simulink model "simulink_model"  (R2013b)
settings: Solver=ode1  StartTime=0.0  StopTime=inf  FixedStep=0.0001  RelTol=1e-3
PostLoadFcn:
  | , if any(exist('dsrtsu_mdlpostloadfcn', 'file') == [2, 3, 6]), try dsrtsu_mdlpostloadfcn('Execute', bdroot); catch fprintf('Error in PostLoadFcn (dsrtsu_mdlpostloadfcn) for model "%s":\n %s\n', bdroot, lasterr); end, end,
libraries: rtilib1103 x8, simulink x4

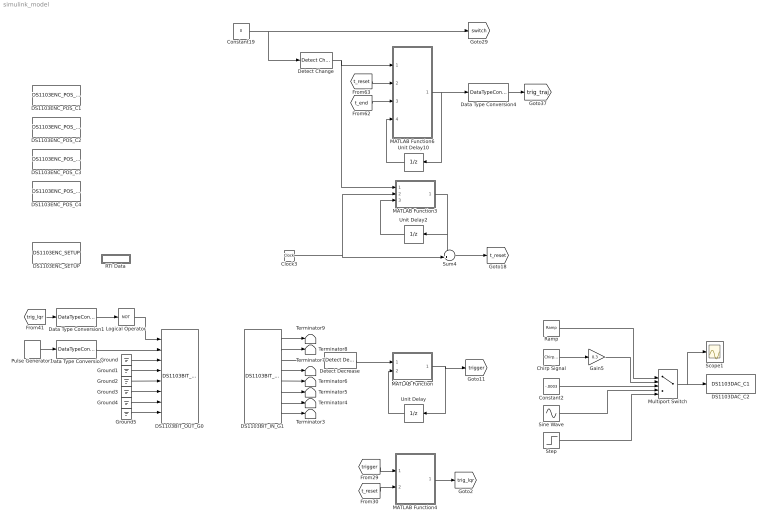
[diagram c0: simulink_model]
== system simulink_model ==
  Chirp Signal : simulink/Sources/Chirp Signal  f1=0.3  T=5  f2=1
  Clock3 : Clock
  Constant19 : Constant  Value=0  OutDataTypeStr=double
  Constant2 : Constant  Value=-.0003  OutDataTypeStr=double
  DS1103BIT_IN_G1 : rtilib1103/DS1103 MASTER PPC/DS1103BIT_IN_G0  GroupNo=1  Reserved1=[]  Reserved2=[]  Reserved3=[]  Reserved4=[]  DialogFcn=gui1103bit_inx  UnitName={ 'DS1103BIT_IN_G'}  UnitValues={ 1 }  DSProperties=struct('RTI',struct('Version',uint32(1),'BlockType',struct('isSLSource',uint8(1),'isSLSink',uint8(0),'isHWSource',uint8(1),'isHWSink',uint8(0),'isSetup',uint8(0),'isInline',uint8(1),'isNonInline',uint8(0),'isInterrupt',uint8(0),'isChannelwise',uint8(0)),'IOBoardType','DS1103MASTER','UnitType','BIT','Identifier','BITIN','DialogType','ML','BlockSet','NONE','SlaveProcessor','NONE'))
  DS1103BIT_OUT_G0 : rtilib1103/DS1103 MASTER PPC/DS1103BIT_OUT_G0  GroupNo=0  InitValue=[0 0 0 0 0 0 0 0]  TermMode=[1 1 1 1 1 1 1 1]  TermValue=[0 0 0 0 0 0 0 0]  Reserved1=[]  Reserved2=[]  Reserved3=[]  Reserved=[]  DialogFcn=gui1103bit_out  UnitName={ 'DS1103BIT_OUT_G'}  UnitValues={ 0 }  DSProperties=struct('RTI',struct('Version',uint32(1),'BlockType',struct('isSLSource',uint8(0),'isSLSink',uint8(1),'isHWSource',uint8(0),'isHWSink',uint8(1),'isSetup',uint8(0),'isInline',uint8(1),'isNonInline',uint8(0),'isInterrupt',uint8(0),'isChannelwise',uint8(0)),'IOBoardType','DS1103MASTER','UnitType','BIT','Identifier','BITOUT','DialogType','ML','BlockSet','NONE','SlaveProcessor','NONE'))
  DS1103DAC_C2 : rtilib1103/DS1103 MASTER PPC/DS1103DAC_C1  ChannelNo=2  InitValue=0  TermMode=1  TermValue=0  Reserved1=[]  Reserved2=[]  Reserved3=[]  Reserved4=[]  DialogFcn=gui1103dac  UnitName={ 'DS1103DAC_C' }  UnitValues={ 2 }  DSProperties=struct('RTI',struct('Version',uint32(1),'BlockType',struct('isSLSource',uint8(0),'isSLSink',uint8(1),'isHWSource',uint8(0),'isHWSink',uint8(1),'isSetup',uint8(0),'isInline',uint8(1),'isNonInline',uint8(0),'isInterrupt',uint8(0),'isChannelwise',uint8(1)),'IOBoardType','DS1103MASTER','UnitType','DAC','Identifier','DAC','DialogType','ML','BlockSet','NONE','SlaveProcessor','NONE'))
  DS1103ENC_POS_C1 : rtilib1103/DS1103 MASTER PPC/DS1103ENC_POS_C1  ChannelNo=1  PosValue=-1024  Reserved1=[]  Reserved2=[]  Reserved3=[]  Reserved4=[]  DialogFcn=gui1103enc_pos  UnitName={ 'DS1103ENC_POS_C' }  UnitValues={ 1 }  DSProperties=struct('RTI',struct('Version',uint32(1),'BlockType',struct('isSLSource',uint8(1),'isSLSink',uint8(0),'isHWSource',uint8(1),'isHWSink',uint8(0),'isSetup',uint8(0),'isInline',uint8(1),'isNonInline',uint8(0),'isInterrupt',uint8(0),'isChannelwise',uint8(1)),'IOBoardType','DS1103MASTER','UnitType','ENC','Identifier','ENCPOSCH','DialogType','ML','BlockSet','NONE','SlaveProcessor','NONE'))
  DS1103ENC_POS_C2 : rtilib1103/DS1103 MASTER PPC/DS1103ENC_POS_C1  ChannelNo=2  PosValue=0  Reserved1=[]  Reserved2=[]  Reserved3=[]  Reserved4=[]  DialogFcn=gui1103enc_pos  UnitName={ 'DS1103ENC_POS_C' }  UnitValues={ 2 }  DSProperties=struct('RTI',struct('Version',uint32(1),'BlockType',struct('isSLSource',uint8(1),'isSLSink',uint8(0),'isHWSource',uint8(1),'isHWSink',uint8(0),'isSetup',uint8(0),'isInline',uint8(1),'isNonInline',uint8(0),'isInterrupt',uint8(0),'isChannelwise',uint8(1)),'IOBoardType','DS1103MASTER','UnitType','ENC','Identifier','ENCPOSCH','DialogType','ML','BlockSet','NONE','SlaveProcessor','NONE'))
  DS1103ENC_POS_C3 : rtilib1103/DS1103 MASTER PPC/DS1103ENC_POS_C1  ChannelNo=3  PosValue=0  Reserved1=[]  Reserved2=[]  Reserved3=[]  Reserved4=[]  DialogFcn=gui1103enc_pos  UnitName={ 'DS1103ENC_POS_C' }  UnitValues={3}  DSProperties=struct('RTI',struct('Version',uint32(1),'BlockType',struct('isSLSource',uint8(1),'isSLSink',uint8(0),'isHWSource',uint8(1),'isHWSink',uint8(0),'isSetup',uint8(0),'isInline',uint8(1),'isNonInline',uint8(0),'isInterrupt',uint8(0),'isChannelwise',uint8(1)),'IOBoardType','DS1103MASTER','UnitType','ENC','Identifier','ENCPOSCH','DialogType','ML','BlockSet','NONE','SlaveProcessor','NONE'))
  DS1103ENC_POS_C4 : rtilib1103/DS1103 MASTER PPC/DS1103ENC_POS_C1  ChannelNo=4  PosValue=0  Reserved1=[]  Reserved2=[]  Reserved3=[]  Reserved4=[]  DialogFcn=gui1103enc_pos  UnitName={ 'DS1103ENC_POS_C' }  UnitValues={ 4 }  DSProperties=struct('RTI',struct('Version',uint32(1),'BlockType',struct('isSLSource',uint8(1),'isSLSink',uint8(0),'isHWSource',uint8(1),'isHWSink',uint8(0),'isSetup',uint8(0),'isInline',uint8(1),'isNonInline',uint8(0),'isInterrupt',uint8(0),'isChannelwise',uint8(1)),'IOBoardType','DS1103MASTER','UnitType','ENC','Identifier','ENCPOSCH','DialogType','ML','BlockSet','NONE','SlaveProcessor','NONE'))
  DS1103ENC_SETUP : rtilib1103/DS1103 MASTER PPC/DS1103ENC_SETUP  EncRange=0  Reserved1=[]  Reserved2=[]  Reserved3=[]  Reserved4=[]  DialogFcn=gui1103enc_setup  UnitName={ 'DS1103ENC_SETUP' }  UnitValues={ [] }  DSProperties=struct('RTI',struct('Version',uint32(1),'BlockType',struct('isSLSource',uint8(0),'isSLSink',uint8(0),'isHWSource',uint8(0),'isHWSink',uint8(0),'isSetup',uint8(0),'isInline',uint8(1),'isNonInline',uint8(0),'isInterrupt',uint8(0),'isChannelwise',uint8(0)),'IOBoardType','DS1103MASTER','UnitType','ENC','Identifier','ENCMASTER','DialogType','ML','BlockSet','NONE','SlaveProcessor','NONE'))
  Data Type Conversion : DataTypeConversion
  Data Type Conversion1 : DataTypeConversion
  Data Type Conversion4 : DataTypeConversion  OutDataTypeStr=boolean
  Detect Change : simulink/Logic and Bit Operations/Detect Change  vinit=0  InputProcessing=Inherited  OutDataTypeStr=boolean
  Detect Decrease : simulink/Logic and Bit Operations/Detect Decrease  vinit=0.0  InputProcessing=Inherited  OutDataTypeStr=boolean
  Gain5 : Gain  Gain=0.3
  Ground{,1..5} (6 alike) : Ground
  Logical Operator : Logic  Operator=NOT  IconShape=distinctive  AllPortsSameDT=off  OutDataTypeStr=boolean
  MATLAB Function : MATLAB Function  TreatAsAtomicUnit=on
  MATLAB Function3 : MATLAB Function  TreatAsAtomicUnit=on
  MATLAB Function4 : MATLAB Function  TreatAsAtomicUnit=on
  MATLAB Function6 : MATLAB Function  TreatAsAtomicUnit=on
  Multiport Switch : MultiPortSwitch  Inputs=5
  Pulse Generator1 : DiscretePulseGenerator  PulseType=Time based  Period=0.001  PulseWidth=10
  RTI Data : Subsystem  Tag=struct('RTIDataServer',struct('RTIDataServerVs','2','RTIModelDescription','struct(''main'',''openloop_model_test_bewegung_3'',''sub'','''',''isMp'',0)'))  LoadFcn="if exist('rtidc'), try,  rtidc('DataHostBlockClbLoad', gcbh); catch, disp(['Warning: ''LoadFcn'' for RTI Data block failed: ' lasterr]); end, end,"
  Ramp : simulink/Sources/Ramp  slope=0.01  start=0  X0=0
  Scope1 : Scope
  Sine Wave : Sin  Amplitude=-0.045  SampleTime=0
  Step : Step  SampleTime=0
  Sum4 : Sum  Inputs=-+|
  Terminator{3..9} (7 alike) : Terminator
  Unit Delay : UnitDelay  InitialCondition=1  SampleTime=-1
  Unit Delay10 : UnitDelay  SampleTime=-1
  Unit Delay2 : UnitDelay  SampleTime=-1
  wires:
  Data Type Conversion/1 -> DS1103BIT_OUT_G0/2
  Pulse Generator1/1 -> Data Type Conversion/1
  [trig_lqr] -> Data Type Conversion1/1
  Data Type Conversion1/1 -> Logical Operator/1
  Logical Operator/1 -> DS1103BIT_OUT_G0/1
  Ground/1 -> DS1103BIT_OUT_G0/3
  Ground5/1 -> DS1103BIT_OUT_G0/8
  Ground1/1 -> DS1103BIT_OUT_G0/4
  Ground3/1 -> DS1103BIT_OUT_G0/6
  Ground2/1 -> DS1103BIT_OUT_G0/5
  Ground4/1 -> DS1103BIT_OUT_G0/7
  Detect Decrease/1 -> MATLAB Function/1(trigger)
  MATLAB Function/1(trigger_set) -> Unit Delay/1, [trigger]
  Unit Delay/1 -> MATLAB Function/2(trigger_set_alt)
  DS1103BIT_IN_G1/3 -> Detect Decrease/1
  [trigger] -> MATLAB Function4/1(trigger)
  MATLAB Function4/1(trigger_lqr) -> [trig_lqr]
  DS1103BIT_IN_G1/2 -> Terminator8/1
  DS1103BIT_IN_G1/1 -> Terminator9/1
  DS1103BIT_IN_G1/4 -> Terminator7/1
  DS1103BIT_IN_G1/8 -> Terminator3/1
  DS1103BIT_IN_G1/5 -> Terminator6/1
  DS1103BIT_IN_G1/6 -> Terminator5/1
  DS1103BIT_IN_G1/7 -> Terminator4/1
  Constant19/1 -> Detect Change/1, [switch]
  Clock3/1 -> Sum4/2, MATLAB Function3/2(time)
  MATLAB Function3/1(time_set) -> Unit Delay2/1, Sum4/1
  Unit Delay2/1 -> MATLAB Function3/3(time_set_old)
  Sum4/1 -> [t_reset]
  Detect Change/1 -> MATLAB Function3/1(trigger), MATLAB Function6/1(trigger)
  MATLAB Function6/1(trigger_set) -> Unit Delay10/1, Data Type Conversion4/1
  Unit Delay10/1 -> MATLAB Function6/4(trigger_set_alt)
  [t_end] -> MATLAB Function6/3(t_end)
  [t_reset] -> MATLAB Function6/2(time)
  Data Type Conversion4/1 -> [trig_traj]
  [t_reset] -> MATLAB Function4/2(t_reset)
  Chirp Signal/1 -> Gain5/1
  Sine Wave/1 -> Multiport Switch/5
  Step/1 -> Multiport Switch/6
  Constant2/1 -> Multiport Switch/4
  Gain5/1 -> Multiport Switch/3
  Ramp/1 -> Multiport Switch/2
  Multiport Switch/1 -> Scope1/1, DS1103DAC_C2/1

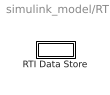
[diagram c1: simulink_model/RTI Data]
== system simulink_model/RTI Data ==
  RTI Data Store : Subsystem  Tag=struct('public',struct('sub',struct('name',{{'openloop_model_test_bewegung_3'}},'data',{{struct('TH',struct('thTaskInfo',struct('taskType',{'TIMER','HWINT','TMRINT','SWINT','GLINT'},'tasksNumOf',{1,0,0,0,0},'srcIds',{{'TIMERA'},{},{},{},{}},'taskNames',{{['Timer Task 1']},{},{},{},{}})),'th_tc',struct('dataType','TASK','taskGroupId','','taskGroupList',{{}},'taskSchedulingPolicy','FCFS','taskType',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

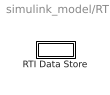
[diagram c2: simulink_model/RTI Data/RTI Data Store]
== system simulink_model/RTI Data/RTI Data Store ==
  RTI Data Store : Subsystem

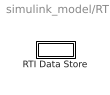
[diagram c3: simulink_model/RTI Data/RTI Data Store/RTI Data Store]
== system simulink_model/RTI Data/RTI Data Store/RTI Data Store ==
  RTI Data Store : Subsystem

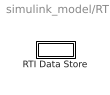
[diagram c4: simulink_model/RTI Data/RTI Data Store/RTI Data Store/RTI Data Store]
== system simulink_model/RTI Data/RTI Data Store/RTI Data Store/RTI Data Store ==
  RTI Data Store : Subsystem

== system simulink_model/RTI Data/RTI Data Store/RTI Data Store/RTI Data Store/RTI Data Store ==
